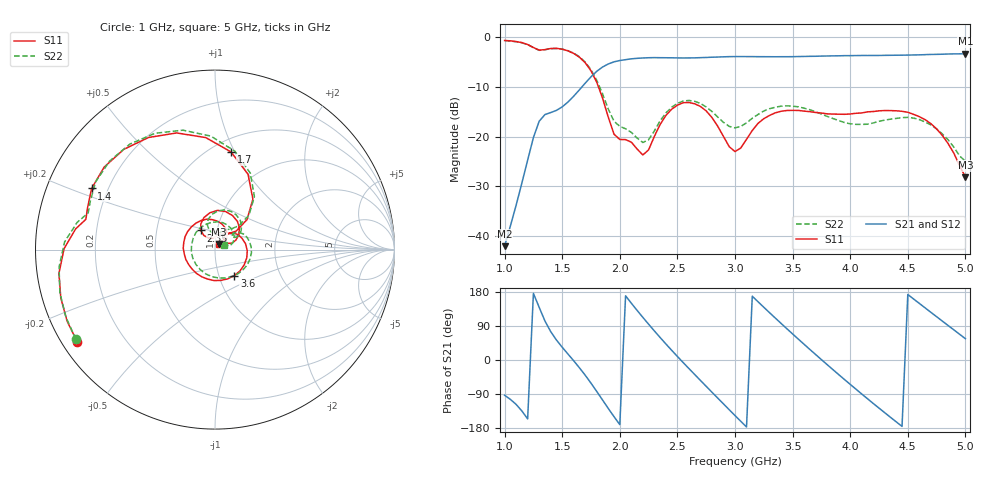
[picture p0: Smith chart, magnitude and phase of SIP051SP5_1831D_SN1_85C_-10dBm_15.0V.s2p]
# GHz  S  dB  R  50
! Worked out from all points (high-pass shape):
!   81 points, 1 GHz to 5 GHz, reference 50 ohm
!   highest |S21| = -3.36 dB at 5 GHz (marker M1); lowest = -42.0 dB at 1 GHz (marker M2)
!   |S21| within 3 dB of the highest: 1.831 GHz to end of sweep
!   lowest |S11| = -28.1 dB at 5 GHz (marker M3), VSWR 1.08, Z = 52.2 + j3.34 ohm
!   |S11| at or under -10 dB: 1.815 GHz to end of sweep
!   |S22| runs from -25.0 to -0.7 dB; largest |S21 - S12| = 0.0019
!   S11 on the Smith chart (normalised r, x): 1 GHz: 0.04, -0.30; 1.4 GHz: 0.14, +0.23; 1.7 GHz: 0.62, +0.97; 2.35 GHz: 0.84, +0.18; 3.6 GHz: 1.18, -0.35; 5 GHz: 1.04, +0.07
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1  -0.69 -146.0  -42.00 -93.1  -41.77 -91.4  -0.70 -147.2
1.25  -2.10 171.5  -20.19 175.9  -20.16 175.6  -2.13 168.8
1.4  -2.30 153.6  -15.17 75.0  -15.15 75.1  -2.33 150.4
1.55  -2.78 120.7  -13.05 15.7  -13.05 15.8  -2.74 117.3
1.7  -5.17 80.7  -9.25 -40.2  -9.24 -40.2  -5.05 78.6
1.85  -12.24 43.1  -6.03 -105.5  -6.01 -105.6  -11.40 45.3
2.05  -20.60 78.0  -4.55 169.3  -4.53 169.4  -18.43 66.8
2.2  -23.69 99.1  -4.21 112.5  -4.19 112.6  -21.18 84.4
2.35  -17.56 126.5  -4.15 59.4  -4.13 59.4  -16.82 107.2
2.6  -13.14 74.7  -4.20 -22.6  -4.19 -22.5  -12.73 67.3
2.8  -16.17 31.7  -4.05 -85.0  -4.04 -85.0  -14.95 35.6
3  -22.99 38.7  -3.93 -146.5  -3.91 -146.6  -18.24 36.7
3.15  -18.78 51.5  -3.93 168.3  -3.93 168.4  -16.32 38.8
3.35  -15.22 10.7  -3.96 110.6  -3.94 110.6  -14.10 13.0
3.6  -14.88 -53.5  -3.90 41.4  -3.90 41.4  -14.29 -35.0
3.7  -15.15 -79.3  -3.86 14.4  -3.84 14.4  -15.03 -57.6
3.85  -15.47 -116.0  -3.78 -25.4  -3.77 -25.4  -16.36 -96.0
4.05  -15.31 -161.2  -3.73 -76.9  -3.72 -77.0  -17.54 -158.4
4.35  -14.77 135.8  -3.67 -151.3  -3.68 -151.3  -16.50 111.2
4.55  -15.53 95.0  -3.60 161.1  -3.60 161.1  -16.28 64.5
4.75  -18.44 57.5  -3.48 114.3  -3.48 114.2  -18.44 27.8
5  -28.14 54.7  -3.36 56.3  -3.35 56.3  -24.98 28.3
